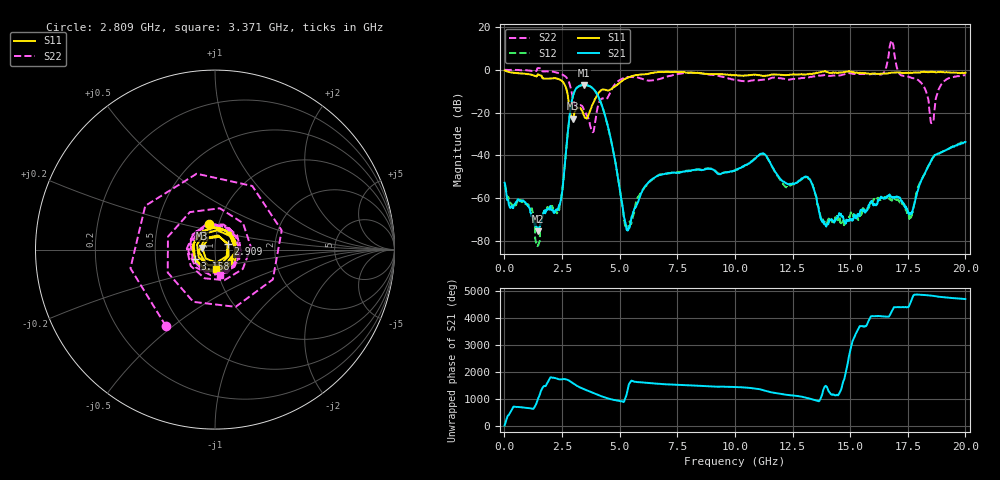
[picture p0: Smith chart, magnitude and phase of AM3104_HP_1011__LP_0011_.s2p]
!Created with skrf (http://scikit-rf.org).
# Hz S RI R 50.0
!freq ReS11 ImS11 ReS21 ImS21 ReS12 ImS12 ReS22 ImS22
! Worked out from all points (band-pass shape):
!   1601 points, 10 MHz to 20 GHz, reference 50 ohm
!   highest |S21| = -7.06 dB at 3.446 GHz (marker M1); lowest = -75.5 dB at 1.459 GHz (marker M2)
!   |S21| within 3 dB of the highest: 3.045 GHz to 3.945 GHz (900.1 MHz wide, 25.8 % of centre)
!   lowest |S11| = -22.9 dB at 2.959 GHz (marker M3), VSWR 1.15, Z = 43.4 + j0.773 ohm
!   |S11| at or under -10 dB: 2.716 GHz to 4.154 GHz (1.438 GHz wide, 41.9 % of centre)
!   |S22| runs from -29.2 to 13.7 dB; largest |S21 - S12| = 0.016
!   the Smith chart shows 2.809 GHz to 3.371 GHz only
!   S11 on the Smith chart (normalised r, x): 2.809 GHz: 0.90, +0.26; 2.909 GHz: 1.15, +0.07; 3.158 GHz: 0.80, -0.08; 3.371 GHz: 0.99, -0.22
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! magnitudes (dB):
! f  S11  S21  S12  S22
! 10 MHz  -0.4  -52.8  -53.8  0.0
! 1.459 GHz  -2.2  -75.5  -82.0  0.8
! 2.396 GHz  -4.6  -63.2  -63.5  -1.7
! 2.809 GHz  -16.7  -23.4  -23.5  -5.9
! 2.909 GHz  -22.3  -15.7  -15.7  -10.0
! 2.959 GHz  -22.9  -12.9  -12.9  -12.7
! 3.158 GHz  -18.2  -8.3  -8.3  -17.3
! 3.346 GHz  -18.7  -7.2  -7.3  -16.7
! 3.371 GHz  -19.1  -7.2  -7.2  -16.9
! 3.446 GHz  -21.2  -7.1  -7.1  -18.6
! 3.821 GHz  -16.3  -8.5  -8.5  -29.1
! 4.32 GHz  -9.3  -19.7  -19.6  -13.7
! 5.332 GHz  -3.8  -75.0  -74.4  -3.3
! 6.682 GHz  -1.1  -49.4  -49.4  -4.5
! 10.01 GHz  -2.7  -47.2  -47.1  -4.8
! 13.34 GHz  -2.0  -53.3  -53.2  -3.3
! 13.97 GHz  -0.9  -73.3  -71.4  -2.6
! 16.68 GHz  -1.6  -59.0  -60.1  7.2
! 17.63 GHz  -1.4  -67.7  -67.9  -3.6
! 18.54 GHz  -0.9  -41.9  -42.1  -24.9
! 18.99 GHz  -1.2  -38.4  -38.4  -6.4
! 20 GHz  -1.4  -33.8  -33.4  -2.5
